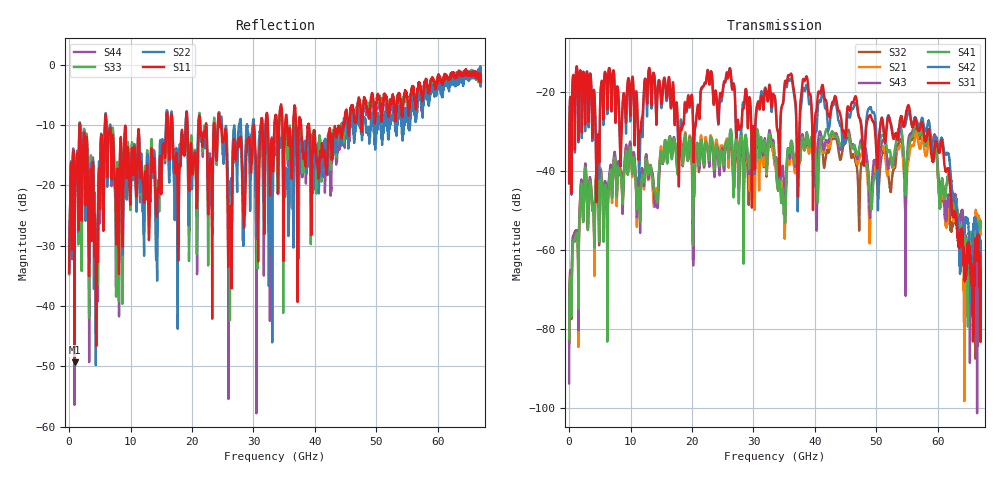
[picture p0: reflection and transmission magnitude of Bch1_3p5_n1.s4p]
!Agilent Technologies,N5247A,US51170199,A.09.90.13
!Agilent N5247A: A.09.90.13
!Date: Wednesday, October 17, 2018 17:33:45
!Correction: S11(Full 4 Port(1,2,3,4))
!S12(Full 4 Port(1,2,3,4))
!S13(Full 4 Port(1,2,3,4))
!S14(Full 4 Port(1,2,3,4))
!S21(Full 4 Port(1,2,3,4))
!S22(Full 4 Port(1,2,3,4))
!S23(Full 4 Port(1,2,3,4))
!S24(Full 4 Port(1,2,3,4))
!S31(Full 4 Port(1,2,3,4))
!S32(Full 4 Port(1,2,3,4))
!S33(Full 4 Port(1,2,3,4))
!S34(Full 4 Port(1,2,3,4))
!S41(Full 4 Port(1,2,3,4))
!S42(Full 4 Port(1,2,3,4))
!S43(Full 4 Port(1,2,3,4))
!S44(Full 4 Port(1,2,3,4))
!S4P File: Measurements: <S11,S12,S13,S14>,
!<S21,S22,S23,S24>,
!<S31,S32,S33,S34>,
!<S41,S42,S43,S44>:
# Hz S  dB  R 50
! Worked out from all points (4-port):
!   6701 points, 10 MHz to 67 GHz, reference 50 ohm
!   strongest paths, dB at 10 MHz, 16.76 GHz, 33.51 GHz, 50.25 GHz, 67 GHz:
!     S31: -43.1, -20.9, -21.8, -36.2, -76.1
!     S42: -43.2, -21.2, -21.2, -50.0, -63.5
!     S41: -81.3, -36.8, -36.5, -36.0, -53.3
!     S43: -93.7, -35.7, -37.5, -41.5, -59.7
!     S21: -83.5, -35.8, -37.8, -40.0, -54.4
!     S32: -82.4, -36.3, -38.4, -46.8, -68.8
!   lowest |S11| = -49.4 dB at 899.9 MHz (marker M1), VSWR 1.01, Z = 49.7 + j0.105 ohm
!   |S11| at or under -10 dB: 6.076 GHz to 15.8 GHz (9.729 GHz wide, 88.9 % of centre); 24.76 GHz to 30.02 GHz (5.259 GHz wide, 19.2 % of centre); 39.05 GHz to 44.61 GHz (5.563 GHz wide, 13.3 % of centre)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
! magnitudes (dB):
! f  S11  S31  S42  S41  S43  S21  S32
! 10 MHz  -34.5  -43.1  -43.2  -81.3  -93.7  -83.5  -82.4
! 899.9 MHz  -49.4  -24.8  -25.3  -57.2  -55.6  -55.6  -57.8
! 4.649 GHz  -32.0  -33.6  -36.2  -41.1  -40.1  -39.9  -41.1
! 6.349 GHz  -12.3  -17.4  -17.2  -47.1  -45.6  -46.0  -47.0
! 26.17 GHz  -25.7  -14.1  -14.0  -30.3  -32.1  -32.6  -32.8
! 55.17 GHz  -7.0  -23.4  -25.0  -34.4  -32.4  -37.8  -34.4
! 67 GHz  -2.8  -76.1  -63.5  -53.3  -59.7  -54.4  -68.8
